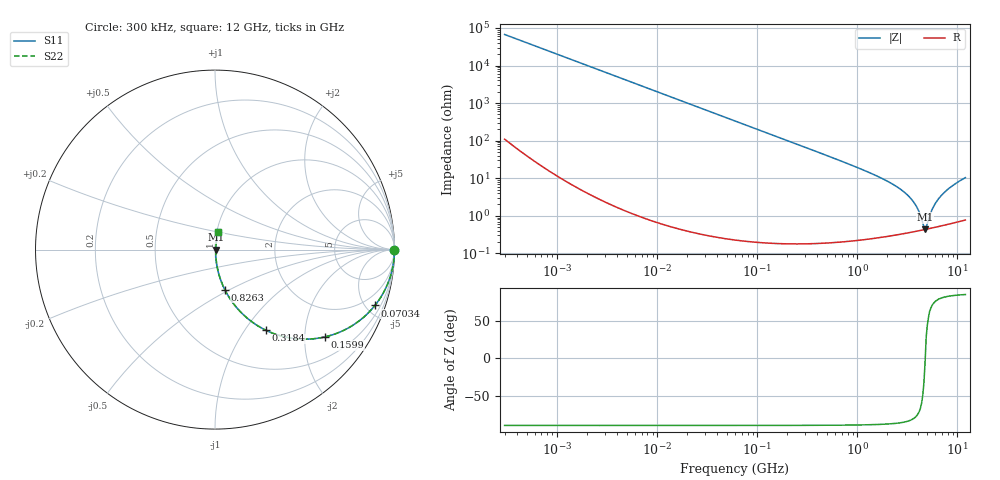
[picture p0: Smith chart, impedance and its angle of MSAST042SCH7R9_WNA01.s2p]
! MSAST042SCH7R9_WNA01  S-PARAMETER MODEL  ( General Type )
! Model Generated by TAIYO YUDEN Corporation (http://www.ty-top.com)
! Version 1.0
! TAIYO YUDEN Control No. 150820
! Copyright(c) 2015 TAIYO YUDEN CO.,LTD. All Rights Reserved.
! Product Description (link to TY-COMPAS)
! https://ds.yuden.co.jp/TYCOMPAS/or/detail?pn=MSAST042SCH7R9BWNA01&u=M
! Products Name : Multilayer Ceramic Capacitors
! Characteristics :
!  Capacitance : 7.9 pF , Rated Voltage : 25V , TCC : CH / C0H
!  Case Size : 0.4 x 0.2 / 0.016 x 0.008 [mm/inch] , Thickness : 0.2 / 0.008 [mm/inch]
!  (Conditions: Temperature = 25 degC , DC Bias Current/Voltage = 0A / 0V)
! External Node Assignments :
!  1  o---| |---o  2
! GND o---------o GND
! Frequency Range : 0.3MHz  -  12000MHz  [ 401 STEP ]
# MHz S RI R 50
! Freq[MHz].  S11 Real  S11 Imag  S21 Real  S21 Imag  S12 Real  S12 Imag  S22 Real  S22 Imag
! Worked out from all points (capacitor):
!   401 points, 300 kHz to 12 GHz, reference 50 ohm
!   read as one part in series: C = 7.9 pF near 316.3 kHz
!   lowest |Z| = 434 mohm at 4.748 GHz (marker M1)
!   series resonance near 4.766 GHz, so ESL is about 140 pH
!   S11 on the Smith chart (normalised r, x): 300 kHz: open; 70.34 MHz: 1.00, -5.73; 159.9 MHz: 1.00, -2.52; 318.4 MHz: 1.00, -1.26; 826.3 MHz: 1.00, -0.47; 12 GHz: 1.02, +0.21
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0.3  1 -0.00149  4.64e-06 0.00149  4.64e-06 0.00149  1 -0.00149
1.769972  0.9999 -0.00878  8.08e-05 0.00878  8.08e-05 0.00878  0.9999 -0.00878
10.44266  0.9973 -0.0517  0.00269 0.0517  0.00269 0.0517  0.9973 -0.0517
27.10171  0.9822 -0.132  0.0178 0.132  0.0178 0.132  0.9822 -0.132
60  0.9184 -0.2734  0.0816 0.2734  0.0816 0.2734  0.9184 -0.2734
70.33673  0.8912 -0.311  0.1088 0.311  0.1088 0.311  0.8912 -0.311
159.8975  0.6131 -0.4863  0.3869 0.4863  0.3869 0.4863  0.6131 -0.4863
318.4019  0.2849 -0.4499  0.7151 0.4499  0.7151 0.4499  0.2849 -0.4499
353.9943  0.2435 -0.4276  0.7565 0.4276  0.7565 0.4276  0.2435 -0.4276
826.3444  0.0548 -0.2232  0.9452 0.2232  0.9452 0.2232  0.0548 -0.2232
2088.533  0.00887 -0.0771  0.9911 0.0771  0.9911 0.0771  0.00887 -0.0771
2795.104  0.00549 -0.047  0.9945 0.047  0.9945 0.047  0.00549 -0.047
3454.93  0.00439 -0.0276  0.9956 0.0276  0.9956 0.0276  0.00439 -0.0276
3944.255  0.00415 -0.0161  0.9959 0.0161  0.9959 0.0161  0.00415 -0.0161
4502.883  0.0042 -0.0049  0.9958 0.0049  0.9958 0.0049  0.0042 -0.0049
4747.894  0.0043 -0.000412  0.9957 0.000412  0.9957 0.000412  0.0043 -0.000412
5006.236  0.00445 0.00443  0.9956 -0.00443  0.9956 -0.00443  0.00445 0.00443
5420.343  0.00476 0.011  0.9952 -0.011  0.9952 -0.011  0.00476 0.011
5868.704  0.00519 0.0182  0.9948 -0.0182  0.9948 -0.0182  0.00519 0.0182
6699.894  0.00621 0.0307  0.9938 -0.0307  0.9938 -0.0307  0.00621 0.0307
8503.825  0.0093 0.0564  0.9907 -0.0564  0.9907 -0.0564  0.0093 0.0564
12000  0.018 0.1007  0.982 -0.1007  0.982 -0.1007  0.018 0.1007
